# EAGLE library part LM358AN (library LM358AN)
Low Power Dual Operational Amplifiers Source: Datasheet
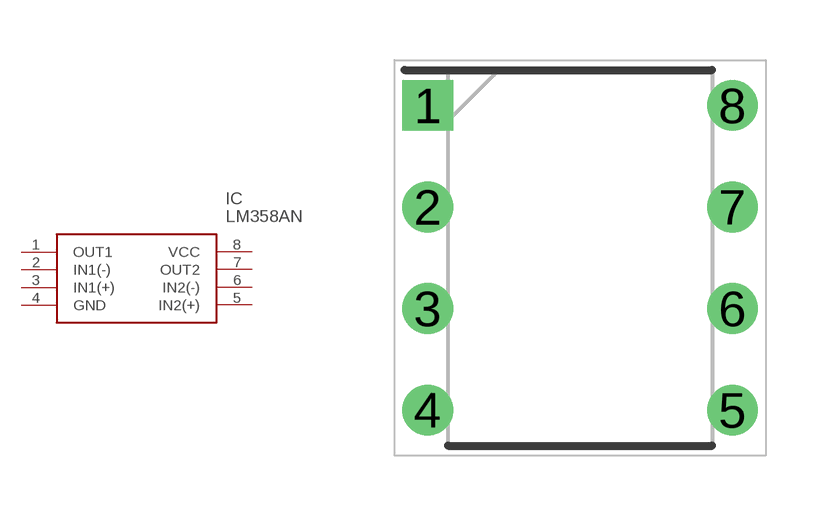
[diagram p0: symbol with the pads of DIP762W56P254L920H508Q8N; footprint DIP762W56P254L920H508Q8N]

Designator prefix IC

## LM358AN (Description: Low Power Dual Operational Amplifiers; Height: 5.08mm; Manufacturer_Name: Texas Instruments; Manufacturer_Part_Number: LM358AN; Mouser_Part_Number: 926-LM358AN; Mouser_Price-Stock: https://www.mouser.co.uk/ProductDetail/Texas-Instruments/LM358AN?qs=QbsRYf82W3GGn0XNxY5ZvQ%3D%3D)  [DIP762W56P254L920H508Q8N]
1  OUT1
2  IN1(-)
3  IN1(+)
4  GND
5  IN2(+)
6  IN2(-)
7  OUT2
8  VCC

## Footprint DIP762W56P254L920H508Q8N (pad centres in mm)
dip
drill 0.76 pad 1.16 square: 1 -3.81,3.81
drill 0.76 pad 1.16: 2 -3.81,1.27; 3 -3.81,-1.27; 4 -3.81,-3.81; 5 3.81,-3.81; 6 3.81,-1.27; 7 3.81,1.27; 8 3.81,3.81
